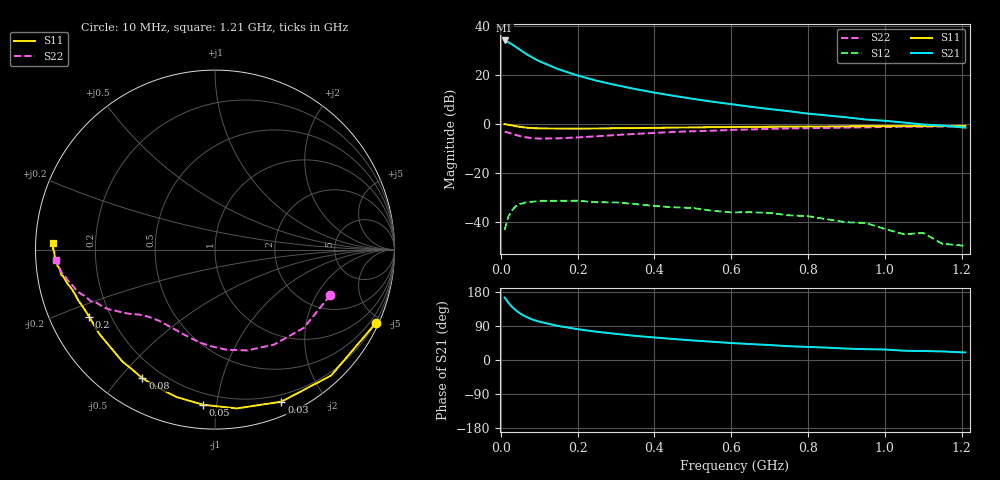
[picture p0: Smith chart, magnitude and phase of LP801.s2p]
!!Date: Tue Nov 09 15:29:30 1999
!  POLYFET RF DEVICES
!  S PARAMETERS FOR
!  LP801
!  VDS=28, IDQ=200mA
# MHZ S MA R 50
! SCATTERING PARAMETERS :
!  FREQ  S11 MAG  S11 ANG  S21 MAG  S21 ANG  S12 MAG  S12 ANG  S22 MAG  S22 ANG
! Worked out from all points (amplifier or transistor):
!   33 points, 10 MHz to 1.21 GHz, reference 50 ohm
!   highest |S21| = 34.1 dB at 10 MHz (marker M1)
!   |S21| within 3 dB of that: start of sweep to 42.5 MHz
!   unconditionally stable (mu >= 1): 741.7 MHz to end of sweep
!   at 60 MHz: K = 0.05, MSG = 30.8 dB, |S12| = -32.4 dB
!   at 450 MHz: K = 0.58, MSG = 22.8 dB, |S12| = -34.2 dB
!   at 1.21 GHz: K = 6.92, MAG = 12.9 dB, |S12| = -50.1 dB
!   S11 on the Smith chart (normalised r, x): 10 MHz: 0.17, -4.60; 30 MHz: 0.13, -1.52; 50 MHz: 0.13, -0.92; 80 MHz: 0.13, -0.58; 200 MHz: 0.12, -0.25; 1.21 GHz: 0.05, +0.02
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10  0.985 -24.5  50.84 165.0  0.00675 75.5  0.6906 -21.6
20  0.9545 -47.3  46.78 151.0  0.01274 62.0  0.6596 -41.3
30  0.9245 -66.4  41.95 139.6  0.0172 51.5  0.6231 -58.3
40  0.8931 -82.2  37.13 130.4  0.02095 42.8  0.5894 -72.3
50  0.8669 -94.4  32.79 123.1  0.02286 33.4  0.5616 -83.4
60  0.849 -104.7  29.02 117.2  0.02389 27.6  0.5388 -92.4
70  0.8312 -112.9  25.86 112.1  0.02546 23.4  0.5236 -99.9
80  0.823 -119.4  23.24 107.8  0.02529 20.1  0.5101 -105.9
90  0.8113 -125.0  21.08 104.3  0.02572 17.3  0.5029 -110.8
100  0.8095 -129.5  19.21 101.3  0.02653 13.1  0.4984 -115.0
150  0.7976 -143.9  13.11 89.6  0.02658 2.2  0.5043 -128.1
200  0.7944 -151.9  9.742 81.3  0.02662 -4.5  0.5267 -134.7
250  0.8024 -156.8  7.614 74.5  0.0248 -10.5  0.5556 -139.3
300  0.8134 -159.7  6.212 69.0  0.02464 -15.8  0.5898 -142.5
350  0.8182 -162.1  5.152 63.7  0.02278 -19.9  0.6215 -145.6
400  0.8268 -164.4  4.349 59.4  0.02083 -21.6  0.6504 -148.5
450  0.8361 -166.0  3.745 55.4  0.01959 -25.4  0.6819 -150.9
550  0.8532 -168.9  2.843 48.2  0.01663 -30.5  0.7209 -155.6
650  0.8674 -170.6  2.237 42.1  0.0155 -24.7  0.7661 -160.1
850  0.8822 -175.1  1.484 32.6  0.01112 -39.4  0.8229 -166.4
1050  0.8962 -179.3  1.061 24.5  0.00548 -37.1  0.8681 -172.4
1210  0.9037 177.5  0.8322 20.1  0.00313 23.1  0.8867 -176.2
